FUNCTION "CENTR. 5  LATERALE DX" : VOID
TITLE =
VERSION : 0.1

BEGIN
NETWORK
TITLE =LETTURA STATUS WORD DA DRIVE
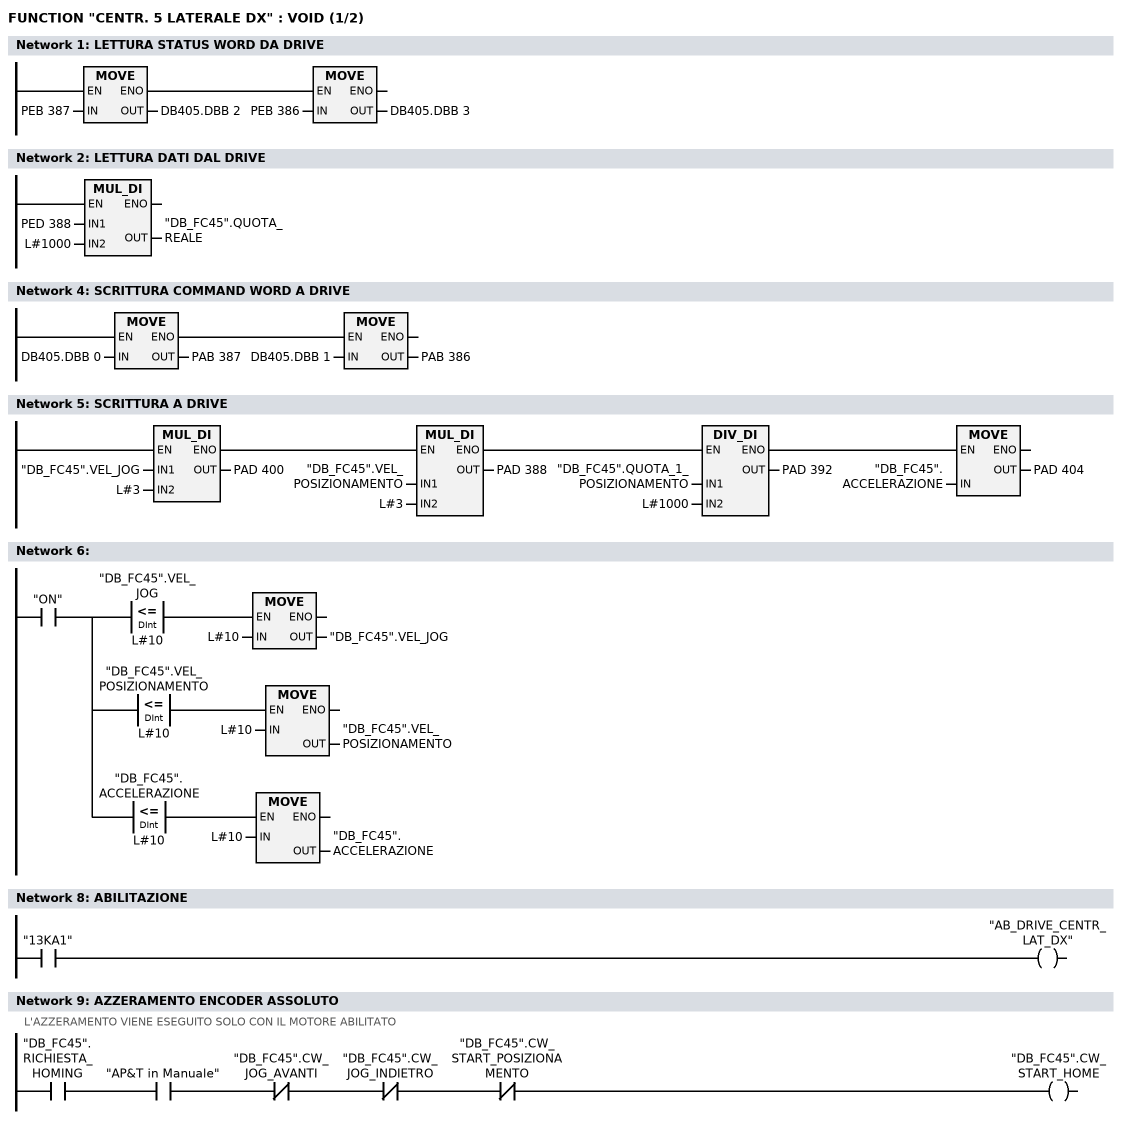
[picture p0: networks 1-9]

      U(    ;
      L     PEB  387;
      T     DB405.DBB    2;
      SET   ;
      SAVE  ;
      CLR   ;
      U     BIE;
      )     ;
      SPBNB _001;
      L     PEB  386;
      T     DB405.DBB    3;
_001: NOP   0;
NETWORK
TITLE =LETTURA DATI DAL DRIVE

      L     PED  388;
      L     L#1000;
      *D    ;
      T     "DB_FC45".QUOTA_REALE;
      NOP   0;
NETWORK
TITLE =

NETWORK
TITLE =SCRITTURA COMMAND WORD A DRIVE

      U(    ;
      L     DB405.DBB    0;
      T     PAB  387;
      SET   ;
      SAVE  ;
      CLR   ;
      U     BIE;
      )     ;
      SPBNB _002;
      L     DB405.DBB    1;
      T     PAB  386;
_002: NOP   0;
NETWORK
TITLE =SCRITTURA A DRIVE

      U(    ;
      U(    ;
      U(    ;
      L     "DB_FC45".VEL_JOG;
      L     L#3;
      *D    ;
      T     PAD  400;
      UN    OV;
      SAVE  ;
      CLR   ;
      U     BIE;
      )     ;
      SPBNB _003;
      L     "DB_FC45".VEL_POSIZIONAMENTO;
      L     L#3;
      *D    ;
      T     PAD  388;
      UN    OV;
      SAVE  ;
      CLR   ;
_003: U     BIE;
      )     ;
      SPBNB _004;
      L     "DB_FC45".QUOTA_1_POSIZIONAMENTO;
      L     L#1000;
      /D    ;
      T     PAD  392;
      UN    OV;
      SAVE  ;
      CLR   ;
_004: U     BIE;
      )     ;
      SPBNB _005;
      L     "DB_FC45".ACCELERAZIONE;
      T     PAD  404;
_005: NOP   0;
NETWORK
TITLE =

      U     "ON";
      =     L      0.0;
      U     L      0.0;
      U(    ;
      L     "DB_FC45".VEL_JOG;
      L     L#10;
      <=D   ;
      )     ;
      SPBNB _006;
      L     L#10;
      T     "DB_FC45".VEL_JOG;
_006: NOP   0;
      U     L      0.0;
      U(    ;
      L     "DB_FC45".VEL_POSIZIONAMENTO;
      L     L#10;
      <=D   ;
      )     ;
      SPBNB _007;
      L     L#10;
      T     "DB_FC45".VEL_POSIZIONAMENTO;
_007: NOP   0;
      U     L      0.0;
      U(    ;
      L     "DB_FC45".ACCELERAZIONE;
      L     L#10;
      <=D   ;
      )     ;
      SPBNB _008;
      L     L#10;
      T     "DB_FC45".ACCELERAZIONE;
_008: NOP   0;
NETWORK
TITLE =

NETWORK
TITLE =ABILITAZIONE

      U     "13KA1";
      =     "AB_DRIVE_CENTR_LAT_DX";
NETWORK
TITLE =AZZERAMENTO ENCODER ASSOLUTO
//L'AZZERAMENTO VIENE ESEGUITO SOLO CON IL MOTORE ABILITATO
      U     "DB_FC45".RICHIESTA_HOMING;
      U     "AP&T in Manuale";
      UN    "DB_FC45".CW_JOG_AVANTI;
      UN    "DB_FC45".CW_JOG_INDIETRO;
      UN    "DB_FC45".CW_START_POSIZIONAMENTO;
      =     "DB_FC45".CW_START_HOME;
NETWORK
TITLE =COMANDI DI JOG
//N.B. VERIFICARE QUOTE EXTRACORSA SOFTWARE
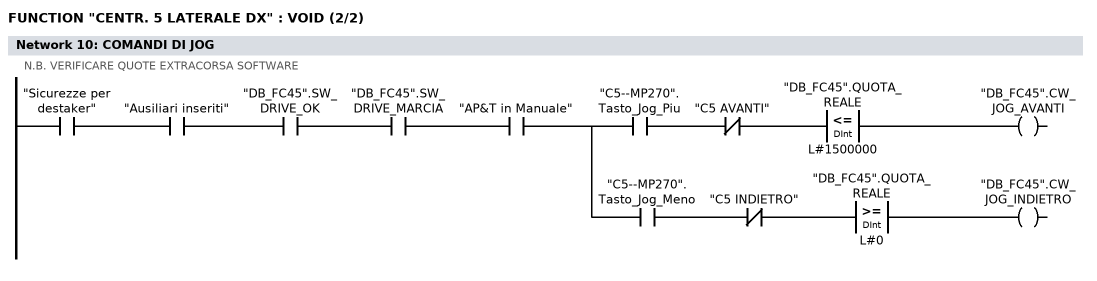
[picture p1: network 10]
      U     "Sicurezze per destaker";
      U     "Ausiliari inseriti";
      U     "DB_FC45".SW_DRIVE_OK;
      U     "DB_FC45".SW_DRIVE_MARCIA;
      U     "AP&T in Manuale";
      =     L      0.0;
      U     L      0.0;
      U     "C5--MP270".Tasto_Jog_Piu;
      UN    "C5 AVANTI";
      U(    ;
      L     "DB_FC45".QUOTA_REALE;
      L     L#1500000;
      <=D   ;
      )     ;
      =     "DB_FC45".CW_JOG_AVANTI;
      U     L      0.0;
      U     "C5--MP270".Tasto_Jog_Meno;
      UN    "C5 INDIETRO";
      U(    ;
      L     "DB_FC45".QUOTA_REALE;
      L     L#0;
      >=D   ;
      )     ;
      =     "DB_FC45".CW_JOG_INDIETRO;
NETWORK
TITLE =Centratore 5: Posizioni

      U     "ON";
      =     L      0.0;
      U     L      0.0;
      U(    ;
      L     "DB_FC45".QUOTA_REALE;
      L     L#100;
      <=D   ;
      )     ;
      U(    ;
      L     "DB_FC45".QUOTA_REALE;
      L     L#-100;
      >=D   ;
      )     ;
      =     "C5: Asse in pos.0";
      U(    ;
      U(    ;
      U     L      0.0;
      SPBNB _009;
      L     "MATRICOLA ATTUALE".C5_Posizione_1;
      L     L#100;
      -D    ;
      T     "CONFRONTI CENTRATORI".C5_Pos_1_Min;
      UN    OV;
      SAVE  ;
      CLR   ;
_009: U     BIE;
      )     ;
      SPBNB _00a;
      L     "MATRICOLA ATTUALE".C5_Posizione_1;
      L     L#200;
      +D    ;
      T     "CONFRONTI CENTRATORI".C5_Pos_1_Max;
      UN    OV;
      SAVE  ;
      CLR   ;
_00a: U     BIE;
      )     ;
      U(    ;
      L     "DB_FC45".QUOTA_REALE;
      L     "CONFRONTI CENTRATORI".C5_Pos_1_Min;
      >=D   ;
      )     ;
      U(    ;
      L     "DB_FC45".QUOTA_REALE;
      L     "CONFRONTI CENTRATORI".C5_Pos_1_Max;
      <=D   ;
      )     ;
      =     "C5: Asse in pos.1";
      U(    ;
      U(    ;
      U     L      0.0;
      SPBNB _00b;
      L     "MATRICOLA ATTUALE".C5_Posizione_2;
      L     L#100;
      -D    ;
      T     "CONFRONTI CENTRATORI".C5_Pos_2_Min;
      UN    OV;
      SAVE  ;
      CLR   ;
_00b: U     BIE;
      )     ;
      SPBNB _00c;
      L     "MATRICOLA ATTUALE".C5_Posizione_2;
      L     L#50000;
      +D    ;
      T     "CONFRONTI CENTRATORI".C5_Pos_2_Max;
      UN    OV;
      SAVE  ;
      CLR   ;
_00c: U     BIE;
      )     ;
      U(    ;
      L     "DB_FC45".QUOTA_REALE;
      L     "CONFRONTI CENTRATORI".C5_Pos_2_Min;
      >=D   ;
      )     ;
      UN    "C5: Asse in pos.3";
      UN    "C5: Asse in pos.4";
      =     "C5: Asse in pos.2";
      U(    ;
      U(    ;
      U     L      0.0;
      SPBNB _00d;
      L     "MATRICOLA ATTUALE".C5_Posizione_3;
      L     L#100;
      -D    ;
      T     "CONFRONTI CENTRATORI".C5_Pos_3_Min;
      UN    OV;
      SAVE  ;
      CLR   ;
_00d: U     BIE;
      )     ;
      SPBNB _00e;
      L     "MATRICOLA ATTUALE".C5_Posizione_3;
      L     L#50000;
      +D    ;
      T     "CONFRONTI CENTRATORI".C5_Pos_3_Max;
      UN    OV;
      SAVE  ;
      CLR   ;
_00e: U     BIE;
      )     ;
      U(    ;
      L     "DB_FC45".QUOTA_REALE;
      L     "CONFRONTI CENTRATORI".C5_Pos_3_Min;
      >=D   ;
      )     ;
      UN    "C5: Asse in pos.4";
      =     "C5: Asse in pos.3";
      U(    ;
      U(    ;
      U     L      0.0;
      SPBNB _00f;
      L     "MATRICOLA ATTUALE".C5_Posizione_4;
      L     L#100;
      -D    ;
      T     "CONFRONTI CENTRATORI".C5_Pos_4_Min;
      UN    OV;
      SAVE  ;
      CLR   ;
_00f: U     BIE;
      )     ;
      SPBNB _010;
      L     "MATRICOLA ATTUALE".C5_Posizione_4;
      L     L#100;
      +D    ;
      T     "CONFRONTI CENTRATORI".C5_Pos_4_Max;
      UN    OV;
      SAVE  ;
      CLR   ;
_010: U     BIE;
      )     ;
      U(    ;
      L     "DB_FC45".QUOTA_REALE;
      L     "CONFRONTI CENTRATORI".C5_Pos_4_Min;
      >=D   ;
      )     ;
      U(    ;
      L     "DB_FC45".QUOTA_REALE;
      L     "CONFRONTI CENTRATORI".C5_Pos_4_Max;
      <=D   ;
      )     ;
      =     "C5: Asse in pos.4";
NETWORK
TITLE =Centratore 5: consenso abilitazione passi
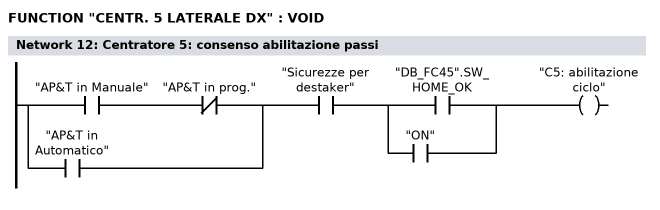
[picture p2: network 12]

      U(    ;
      U     "AP&T in Manuale";
      UN    "AP&T in prog.";
      O     "AP&T in Automatico";
      )     ;
      U     "Sicurezze per destaker";
      U(    ;
      O     "DB_FC45".SW_HOME_OK;
      O     "ON";
      )     ;
      =     "C5: abilitazione ciclo";
NETWORK
TITLE =Centratore 5: comando avvicinamento  (centraggi aperti)

      U(    ;
      U(    ;
      O     "Comando apre centraggi";
      O     "C5--MP270".Tasto_Indietro;
      O     ;
      U     "Apertura centratori";
      U(    ;
      O     "Centratori a riposo";
      O     "Centratori tutti chiusi";
      )     ;
      )     ;
      UN    "C5: Asse in pos.1";
      UN    "C5: comando arrivo";
      UN    "C5: comando a riposo";
      U     "C5: abilitazione ciclo";
      L     S5T#100MS;
      SE    T    194;
      NOP   0;
      NOP   0;
      NOP   0;
      U     T    194;
      )     ;
      S     "C5: comando avvicinam";
      U(    ;
      O     "C5: Asse in pos.1";
      O(    ;
      U(    ;
      O     "Ripristino centratori";
      O     "Comando riposo centraggi";
      O     "C5--MP270".Tasto_Riposo;
      )     ;
      FP    "C5: one shot 1";
      )     ;
      )     ;
      R     "C5: comando avvicinam";
      NOP   0;
NETWORK
TITLE =Centratore 5: comando arrivo (centraggi chiusi)

      U(    ;
      U(    ;
      O     "Comando chiude centraggi";
      O     "C5--MP270".Tasto_Avanti;
      O     ;
      U     "Chiusura centratori";
      U(    ;
      O     "Centratori tutti aperti";
      O     "Centratori a riposo";
      )     ;
      )     ;
      UN    "C5: Asse in pos.4";
      UN    "C5: comando avvicinam";
      UN    "C5: comando a riposo";
      U     "C5: abilitazione ciclo";
      L     S5T#100MS;
      SE    T    195;
      NOP   0;
      NOP   0;
      NOP   0;
      U     T    195;
      )     ;
      S     "C5: comando arrivo";
      U(    ;
      O     "C5: Asse in pos.4";
      O(    ;
      U(    ;
      O     "Ripristino centratori";
      O     "Comando riposo centraggi";
      O     "C5--MP270".Tasto_Riposo;
      )     ;
      FP    "C5: one shot 2";
      )     ;
      )     ;
      R     "C5: comando arrivo";
      NOP   0;
NETWORK
TITLE =Centratore 5: comando automatico centraggi a riposo

      U(    ;
      U(    ;
      O     "Comando riposo centraggi";
      O     "C5--MP270".Tasto_Riposo;
      )     ;
      UN    "C5: Asse in pos.0";
      UN    "C5: comando avvicinam";
      UN    "C5: comando arrivo";
      U     "C5: abilitazione ciclo";
      L     S5T#100MS;
      SE    T    196;
      NOP   0;
      NOP   0;
      NOP   0;
      U     T    196;
      )     ;
      S     "C5: comando a riposo";
      U(    ;
      O     "C5: Asse in pos.0";
      O(    ;
      U     "Ripristino centratori";
      FP    "C5: one shot 3";
      )     ;
      )     ;
      R     "C5: comando a riposo";
      NOP   0;
NETWORK
TITLE =Centratore 5: quote impostate per posizioni

      U     "ON";
      =     L      0.0;
      U(    ;
      U(    ;
      U     L      0.0;
      U     "C5: comando a riposo";
      UN    "C5: Asse in pos.0";
      SPBNB _011;
      L     0;
      T     "DB_FC45".QUOTA_1_POSIZIONAMENTO;
      SET   ;
      SAVE  ;
      CLR   ;
_011: U     BIE;
      )     ;
      SPBNB _012;
      L     L#150;
      T     "DB_FC45".VEL_POSIZIONAMENTO;
      SET   ;
      SAVE  ;
      CLR   ;
_012: U     BIE;
      )     ;
      SPBNB _013;
      L     L#1000;
      T     "DB_FC45".ACCELERAZIONE;
      SET   ;
      SAVE  ;
      CLR   ;
_013: U     BIE;
      =     "C5: Quote pronte pos.0";
      U(    ;
      U(    ;
      U     L      0.0;
      U     "C5: comando avvicinam";
      UN    "C5: Asse in pos.1";
      SPBNB _014;
      L     "MATRICOLA ATTUALE".C5_Posizione_1;
      T     "DB_FC45".QUOTA_1_POSIZIONAMENTO;
      SET   ;
      SAVE  ;
      CLR   ;
_014: U     BIE;
      )     ;
      SPBNB _015;
      L     "MATRICOLA ATTUALE".C5_Velocita_1;
      T     "DB_FC45".VEL_POSIZIONAMENTO;
      SET   ;
      SAVE  ;
      CLR   ;
_015: U     BIE;
      )     ;
      SPBNB _016;
      L     "MATRICOLA ATTUALE".C5_Accell_1;
      T     "DB_FC45".ACCELERAZIONE;
      SET   ;
      SAVE  ;
      CLR   ;
_016: U     BIE;
      =     "C5: Quote pronte pos.1";
      U     L      0.0;
      U     "C5: comando arrivo";
      =     L      0.1;
      U(    ;
      U(    ;
      U     L      0.1;
      UN    "C5: Asse in pos.2";
      SPBNB _017;
      L     "MATRICOLA ATTUALE".C5_Posizione_4;
      T     "DB_FC45".QUOTA_1_POSIZIONAMENTO;
      SET   ;
      SAVE  ;
      CLR   ;
_017: U     BIE;
      )     ;
      SPBNB _018;
      L     "MATRICOLA ATTUALE".C5_Velocita_2;
      T     "DB_FC45".VEL_POSIZIONAMENTO;
      SET   ;
      SAVE  ;
      CLR   ;
_018: U     BIE;
      )     ;
      SPBNB _019;
      L     "MATRICOLA ATTUALE".C5_Accell_2;
      T     "DB_FC45".ACCELERAZIONE;
      SET   ;
      SAVE  ;
      CLR   ;
_019: U     BIE;
      S     "C5: Quote pronte pos.2";
      U     L      0.1;
      U     "C5: Quote pronte pos.2";
      UN    "C5: Reset start pos.2";
      L     S5T#1S;
      SE    "C5: ritardo P2";
      NOP   0;
      NOP   0;
      NOP   0;
      U     "C5: ritardo P2";
      S     "C5: Reset start pos.2";
      R     "C5: Quote pronte pos.2";
      U     L      0.0;
      U     "C5: comando arrivo";
      =     L      0.1;
      U(    ;
      U(    ;
      U(    ;
      U     L      0.1;
      U     "C5: Asse in pos.2";
      UN    "C5: Asse in pos.3";
      SPBNB _01a;
      L     "MATRICOLA ATTUALE".C5_Posizione_4;
      T     "DB_FC45".QUOTA_1_POSIZIONAMENTO;
      SET   ;
      SAVE  ;
      CLR   ;
_01a: U     BIE;
      )     ;
      SPBNB _01b;
      L     "MATRICOLA ATTUALE".C5_Velocita_3;
      T     "DB_FC45".VEL_POSIZIONAMENTO;
      SET   ;
      SAVE  ;
      CLR   ;
_01b: U     BIE;
      )     ;
      SPBNB _01c;
      L     "MATRICOLA ATTUALE".C5_Accell_3;
      T     "DB_FC45".ACCELERAZIONE;
      SET   ;
      SAVE  ;
      CLR   ;
_01c: U     BIE;
      )     ;
      U     "C5: Reset start pos.2";
      S     "C5: Quote pronte pos.3";
      R     "C5: Reset start pos.2";
      U     L      0.1;
      U     "C5: Quote pronte pos.3";
      UN    "C5: Reset start pos.2";
      L     S5T#500MS;
      SE    "C5: ritardo P3";
      NOP   0;
      NOP   0;
      NOP   0;
      U     "C5: ritardo P3";
      S     "C5: Reset start pos.3";
      R     "C5: Quote pronte pos.3";
      U     L      0.0;
      U     "C5: comando arrivo";
      =     L      0.1;
      U(    ;
      U(    ;
      U(    ;
      U     L      0.1;
      U     "C5: Asse in pos.3";
      UN    "C5: Asse in pos.4";
      SPBNB _01d;
      L     "MATRICOLA ATTUALE".C5_Posizione_4;
      T     "DB_FC45".QUOTA_1_POSIZIONAMENTO;
      SET   ;
      SAVE  ;
      CLR   ;
_01d: U     BIE;
      )     ;
      SPBNB _01e;
      L     "MATRICOLA ATTUALE".C5_Velocita_4;
      T     "DB_FC45".VEL_POSIZIONAMENTO;
      SET   ;
      SAVE  ;
      CLR   ;
_01e: U     BIE;
      )     ;
      SPBNB _01f;
      L     "MATRICOLA ATTUALE".C5_Accell_4;
      T     "DB_FC45".ACCELERAZIONE;
      SET   ;
      SAVE  ;
      CLR   ;
_01f: U     BIE;
      )     ;
      U     "C5: Reset start pos.3";
      S     "C5: Quote pronte pos.4";
      R     "C5: Reset start pos.3";
      U     L      0.1;
      U     "C5: Quote pronte pos.4";
      L     S5T#500MS;
      SE    "C5: ritardo P4";
      NOP   0;
      NOP   0;
      NOP   0;
      U     "C5: ritardo P4";
      S     "C5: Reset start pos.4";
      R     "C5: Quote pronte pos.4";
NETWORK
TITLE =Centratore 5: reset impostate
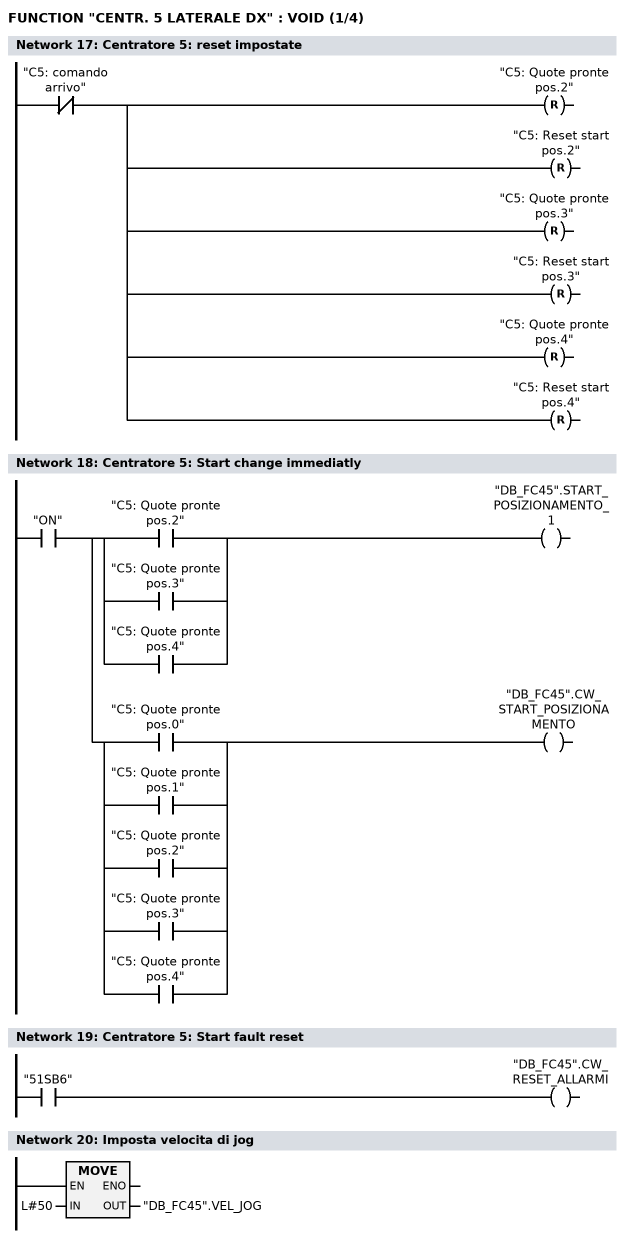
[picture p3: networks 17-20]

      UN    "C5: comando arrivo";
      R     "C5: Quote pronte pos.2";
      R     "C5: Reset start pos.2";
      R     "C5: Quote pronte pos.3";
      R     "C5: Reset start pos.3";
      R     "C5: Quote pronte pos.4";
      R     "C5: Reset start pos.4";
NETWORK
TITLE =Centratore 5: Start change immediatly

      U     "ON";
      =     L      0.0;
      U     L      0.0;
      U(    ;
      O     "C5: Quote pronte pos.2";
      O     "C5: Quote pronte pos.3";
      O     "C5: Quote pronte pos.4";
      )     ;
      =     "DB_FC45".START_POSIZIONAMENTO_1;
      U     L      0.0;
      U(    ;
      O     "C5: Quote pronte pos.0";
      O     "C5: Quote pronte pos.1";
      O     "C5: Quote pronte pos.2";
      O     "C5: Quote pronte pos.3";
      O     "C5: Quote pronte pos.4";
      )     ;
      =     "DB_FC45".CW_START_POSIZIONAMENTO;
NETWORK
TITLE =Centratore 5: Start fault reset

      U     "51SB6";
      =     "DB_FC45".CW_RESET_ALLARMI;
NETWORK
TITLE =Imposta velocita di jog

      L     L#50;
      T     "DB_FC45".VEL_JOG;
      NOP   0;
NETWORK
TITLE =Centratore 5: Drive Enable ok
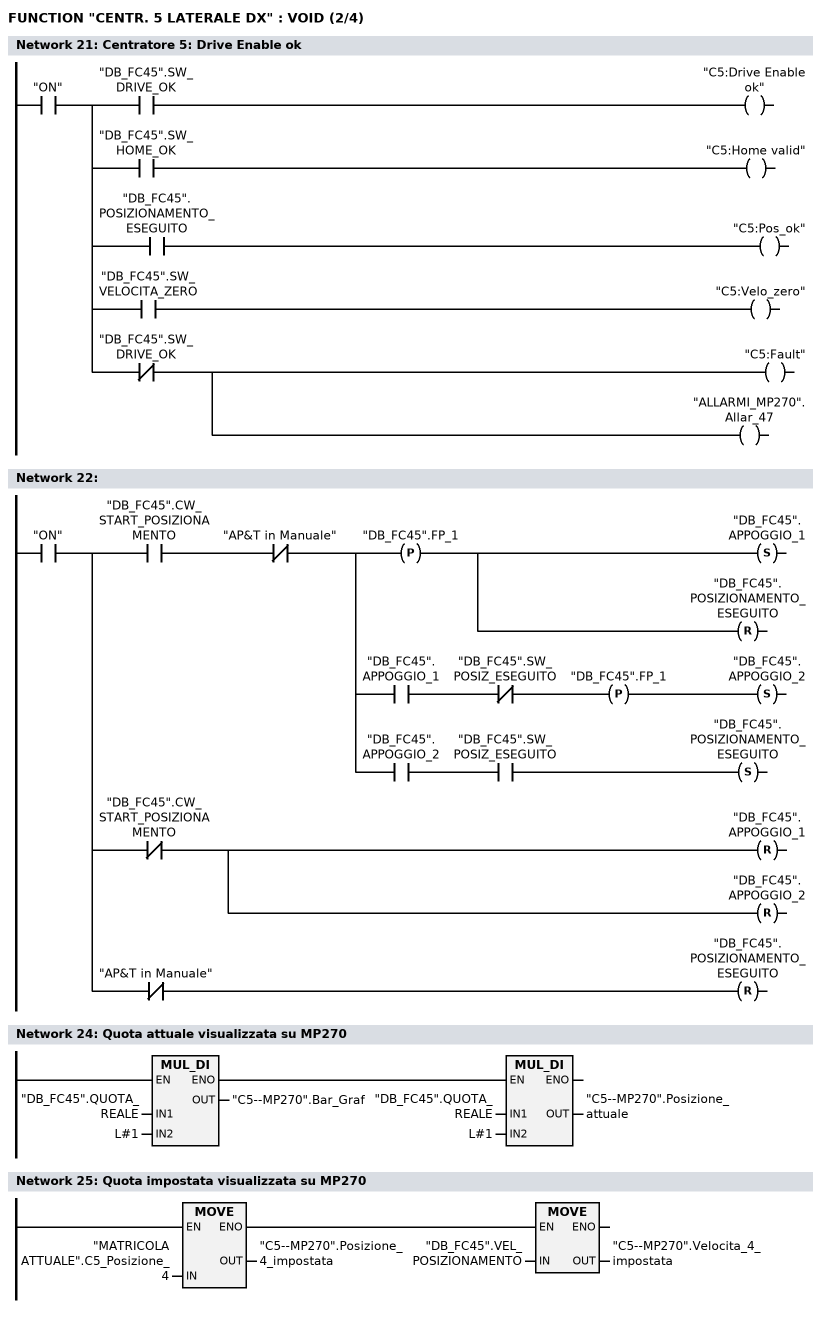
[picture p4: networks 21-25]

      U     "ON";
      =     L      0.0;
      U     L      0.0;
      U     "DB_FC45".SW_DRIVE_OK;
      =     "C5:Drive Enable ok";
      U     L      0.0;
      U     "DB_FC45".SW_HOME_OK;
      =     "C5:Home valid";
      U     L      0.0;
      U     "DB_FC45".POSIZIONAMENTO_ESEGUITO;
      =     "C5:Pos_ok";
      U     L      0.0;
      U     "DB_FC45".SW_VELOCITA_ZERO;
      =     "C5:Velo_zero";
      U     L      0.0;
      UN    "DB_FC45".SW_DRIVE_OK;
      =     "C5:Fault";
      =     "ALLARMI_MP270".Allar_47;
NETWORK
TITLE =

      U     "ON";
      =     L      0.0;
      U     L      0.0;
      U     "DB_FC45".CW_START_POSIZIONAMENTO;
      UN    "AP&T in Manuale";
      =     L      0.1;
      U     L      0.1;
      FP    "DB_FC45".FP_1;
      S     "DB_FC45".APPOGGIO_1;
      R     "DB_FC45".POSIZIONAMENTO_ESEGUITO;
      U     L      0.1;
      U     "DB_FC45".APPOGGIO_1;
      UN    "DB_FC45".SW_POSIZ_ESEGUITO;
      FP    "DB_FC45".FP_1;
      S     "DB_FC45".APPOGGIO_2;
      U     L      0.1;
      U     "DB_FC45".APPOGGIO_2;
      U     "DB_FC45".SW_POSIZ_ESEGUITO;
      S     "DB_FC45".POSIZIONAMENTO_ESEGUITO;
      U     L      0.0;
      UN    "DB_FC45".CW_START_POSIZIONAMENTO;
      R     "DB_FC45".APPOGGIO_1;
      R     "DB_FC45".APPOGGIO_2;
      U     L      0.0;
      UN    "AP&T in Manuale";
      R     "DB_FC45".POSIZIONAMENTO_ESEGUITO;
NETWORK
TITLE =

NETWORK
TITLE =Quota attuale visualizzata su MP270

      U(    ;
      L     "DB_FC45".QUOTA_REALE;
      L     L#1;
      *D    ;
      T     "C5--MP270".Bar_Graf;
      UN    OV;
      SAVE  ;
      CLR   ;
      U     BIE;
      )     ;
      SPBNB _020;
      L     "DB_FC45".QUOTA_REALE;
      L     L#1;
      *D    ;
      T     "C5--MP270".Posizione_attuale;
_020: NOP   0;
NETWORK
TITLE =Quota impostata visualizzata su MP270

      U(    ;
      L     "MATRICOLA ATTUALE".C5_Posizione_4;
      T     "C5--MP270".Posizione_4_impostata;
      SET   ;
      SAVE  ;
      CLR   ;
      U     BIE;
      )     ;
      SPBNB _021;
      L     "DB_FC45".VEL_POSIZIONAMENTO;
      T     "C5--MP270".Velocita_4_impostata;
_021: NOP   0;
NETWORK
TITLE =Visualizza FC su MP270
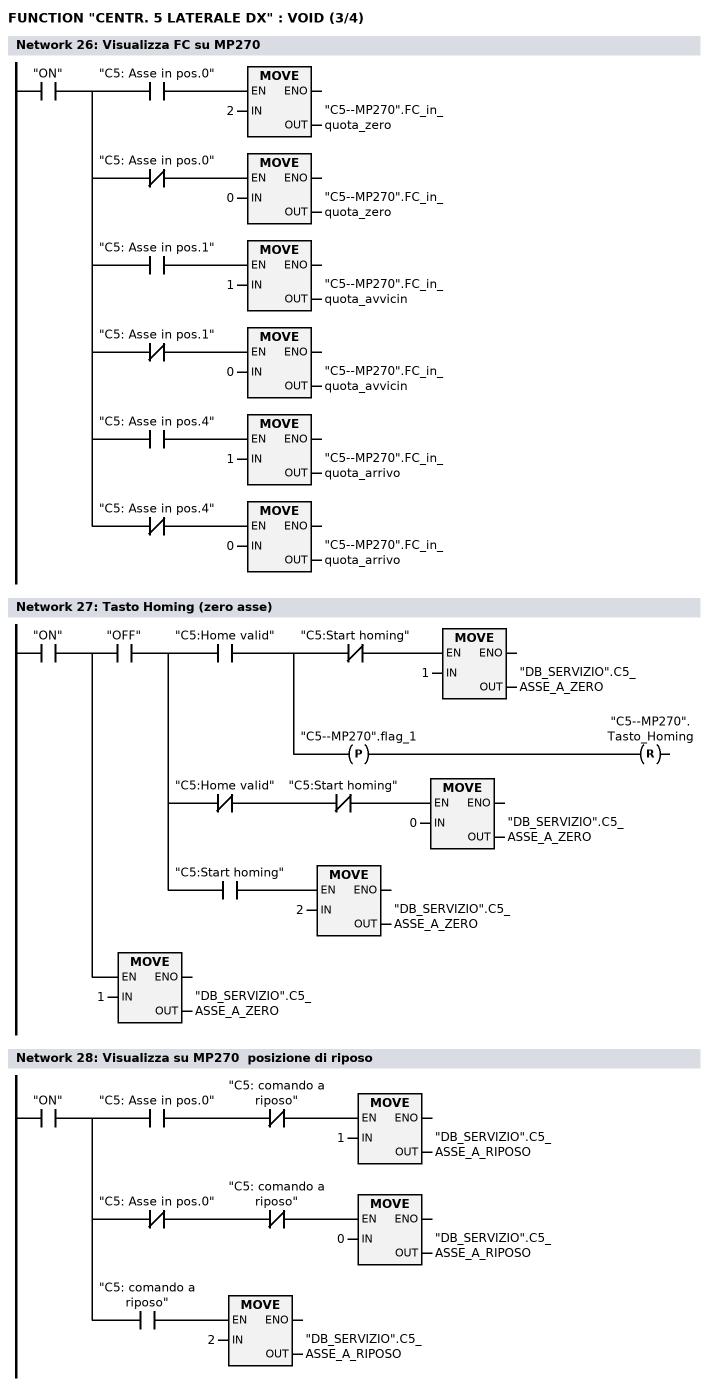
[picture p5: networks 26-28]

      U     "ON";
      =     L      0.0;
      U     L      0.0;
      U     "C5: Asse in pos.0";
      SPBNB _022;
      L     2;
      T     "C5--MP270".FC_in_quota_zero;
_022: NOP   0;
      U     L      0.0;
      UN    "C5: Asse in pos.0";
      SPBNB _023;
      L     0;
      T     "C5--MP270".FC_in_quota_zero;
_023: NOP   0;
      U     L      0.0;
      U     "C5: Asse in pos.1";
      SPBNB _024;
      L     1;
      T     "C5--MP270".FC_in_quota_avvicin;
_024: NOP   0;
      U     L      0.0;
      UN    "C5: Asse in pos.1";
      SPBNB _025;
      L     0;
      T     "C5--MP270".FC_in_quota_avvicin;
_025: NOP   0;
      U     L      0.0;
      U     "C5: Asse in pos.4";
      SPBNB _026;
      L     1;
      T     "C5--MP270".FC_in_quota_arrivo;
_026: NOP   0;
      U     L      0.0;
      UN    "C5: Asse in pos.4";
      SPBNB _027;
      L     0;
      T     "C5--MP270".FC_in_quota_arrivo;
_027: NOP   0;
NETWORK
TITLE =Tasto Homing (zero asse)

      U     "ON";
      =     L      0.0;
      U     L      0.0;
      U     "OFF";
      =     L      0.1;
      U     L      0.1;
      U     "C5:Home valid";
      =     L      0.2;
      U     L      0.2;
      UN    "C5:Start homing";
      SPBNB _028;
      L     1;
      T     "DB_SERVIZIO".C5_ASSE_A_ZERO;
_028: NOP   0;
      U     L      0.2;
      FP    "C5--MP270".flag_1;
      R     "C5--MP270".Tasto_Homing;
      U     L      0.1;
      UN    "C5:Home valid";
      UN    "C5:Start homing";
      SPBNB _029;
      L     0;
      T     "DB_SERVIZIO".C5_ASSE_A_ZERO;
_029: NOP   0;
      U     L      0.1;
      U     "C5:Start homing";
      SPBNB _02a;
      L     2;
      T     "DB_SERVIZIO".C5_ASSE_A_ZERO;
_02a: NOP   0;
      U     L      0.0;
      SPBNB _02b;
      L     1;
      T     "DB_SERVIZIO".C5_ASSE_A_ZERO;
_02b: NOP   0;
NETWORK
TITLE =Visualizza su MP270  posizione di riposo

      U     "ON";
      =     L      0.0;
      U     L      0.0;
      U     "C5: Asse in pos.0";
      UN    "C5: comando a riposo";
      SPBNB _02c;
      L     1;
      T     "DB_SERVIZIO".C5_ASSE_A_RIPOSO;
_02c: NOP   0;
      U     L      0.0;
      UN    "C5: Asse in pos.0";
      UN    "C5: comando a riposo";
      SPBNB _02d;
      L     0;
      T     "DB_SERVIZIO".C5_ASSE_A_RIPOSO;
_02d: NOP   0;
      U     L      0.0;
      U     "C5: comando a riposo";
      SPBNB _02e;
      L     2;
      T     "DB_SERVIZIO".C5_ASSE_A_RIPOSO;
_02e: NOP   0;
NETWORK
TITLE =Visualizza su MP270  posizione di avvicinamento
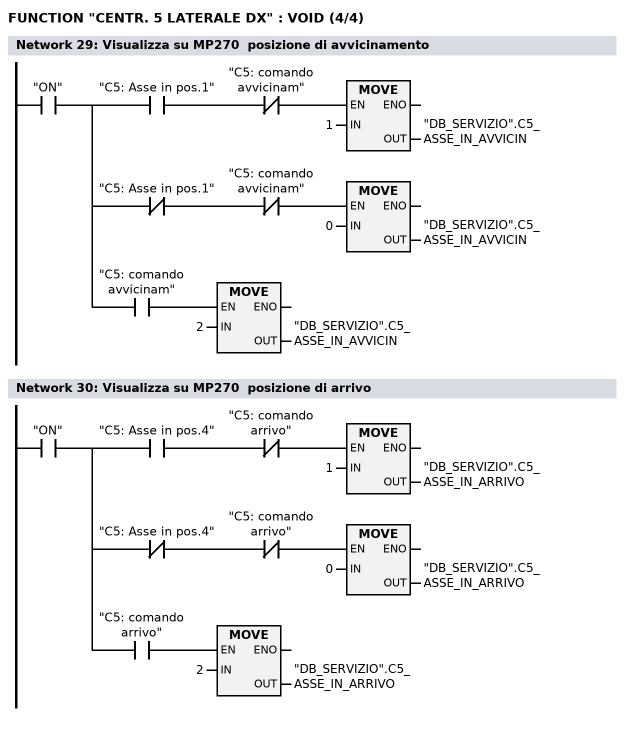
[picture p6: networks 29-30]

      U     "ON";
      =     L      0.0;
      U     L      0.0;
      U     "C5: Asse in pos.1";
      UN    "C5: comando avvicinam";
      SPBNB _02f;
      L     1;
      T     "DB_SERVIZIO".C5_ASSE_IN_AVVICIN;
_02f: NOP   0;
      U     L      0.0;
      UN    "C5: Asse in pos.1";
      UN    "C5: comando avvicinam";
      SPBNB _030;
      L     0;
      T     "DB_SERVIZIO".C5_ASSE_IN_AVVICIN;
_030: NOP   0;
      U     L      0.0;
      U     "C5: comando avvicinam";
      SPBNB _031;
      L     2;
      T     "DB_SERVIZIO".C5_ASSE_IN_AVVICIN;
_031: NOP   0;
NETWORK
TITLE =Visualizza su MP270  posizione di arrivo

      U     "ON";
      =     L      0.0;
      U     L      0.0;
      U     "C5: Asse in pos.4";
      UN    "C5: comando arrivo";
      SPBNB _032;
      L     1;
      T     "DB_SERVIZIO".C5_ASSE_IN_ARRIVO;
_032: NOP   0;
      U     L      0.0;
      UN    "C5: Asse in pos.4";
      UN    "C5: comando arrivo";
      SPBNB _033;
      L     0;
      T     "DB_SERVIZIO".C5_ASSE_IN_ARRIVO;
_033: NOP   0;
      U     L      0.0;
      U     "C5: comando arrivo";
      SPBNB _034;
      L     2;
      T     "DB_SERVIZIO".C5_ASSE_IN_ARRIVO;
_034: NOP   0;
END_FUNCTION

